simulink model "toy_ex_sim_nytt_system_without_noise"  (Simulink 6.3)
settings: Solver=ode4  StartTime=0.0  StopTime=simtid  FixedStep=.05  RelTol=1e-5
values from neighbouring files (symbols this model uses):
  alpha = -0.9    [bounds.m]    (also in real_ex_linkomb_W_and_DP.m = 1; real_ex_linkomb_W_and_RHOT.m = -0.2; real_ex_without_noise_z_30.m = -6:0.01:4; toy_ex_nytt_system.m)
  den_G1 = [-1 1]    [bounds.m]    (also in toy_ex_nytt_system.m; toy_ex_nytt_system_without_noise.m; toy_ex_nytt_system_with_disturbance.m; toy_ex_nytt_system_with_measure_noise.m)
  den_G2 = [-1 1]    [bounds.m]    (also in toy_ex_nytt_system.m; toy_ex_nytt_system_without_noise.m; toy_ex_nytt_system_with_disturbance.m; toy_ex_nytt_system_with_measure_noise.m)
  K_indre = 10    [real_ex_linkomb_W_and_DP.m]    (also in real_ex_linkomb_W_and_RHOT.m = 5; toy_ex_nytt_system.m = 50; toy_ex_nytt_system_without_noise.m = 20; toy_ex_nytt_system_with_disturbance.m = 50)
  K_ytre = 0.01    [real_ex_linkomb_W_and_DP.m]    (also in real_ex_linkomb_W_and_RHOT.m; toy_ex_nytt_system.m = 0.1; toy_ex_nytt_system_without_noise.m = 0.1; toy_ex_nytt_system_with_disturbance.m = 0.1)
  num_G1 = 5*[-1.5 1]    [bounds.m]    (also in toy_ex_nytt_system.m; toy_ex_nytt_system_without_noise.m; toy_ex_nytt_system_with_disturbance.m; toy_ex_nytt_system_with_measure_noise.m)
  num_G2 = 5*[-0.5 1]    [bounds.m]    (also in toy_ex_nytt_system.m; toy_ex_nytt_system_without_noise.m; toy_ex_nytt_system_with_disturbance.m; toy_ex_nytt_system_with_measure_noise.m)
  Ti = 100    [real_ex_linkomb_W_and_DP.m]    (also in real_ex_linkomb_W_and_RHOT.m = 100000; toy_ex_nytt_system.m = 10; toy_ex_nytt_system_without_noise.m = 10; toy_ex_nytt_system_with_disturbance.m = 10)

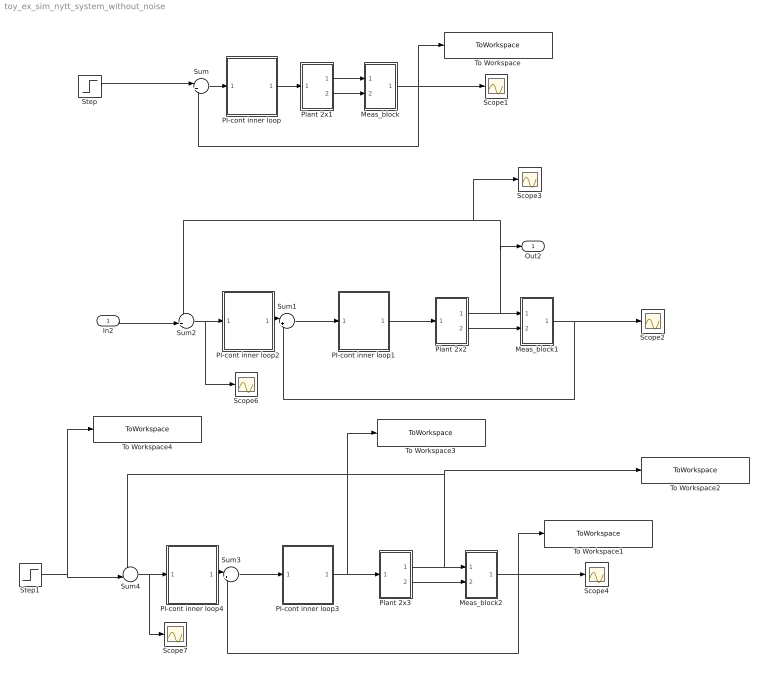
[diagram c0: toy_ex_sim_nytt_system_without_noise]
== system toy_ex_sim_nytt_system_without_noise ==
  In2 : Inport
  Meas_block : Subsystem
  Meas_block1 : Subsystem
  Meas_block2 : Subsystem
  PI-cont inner loop : Subsystem
  PI-cont inner loop1 : Subsystem
  PI-cont inner loop2 : Subsystem
  PI-cont inner loop3 : Subsystem
  PI-cont inner loop4 : Subsystem
  Plant 2x1 : Subsystem
  Plant 2x2 : Subsystem
  Plant 2x3 : Subsystem
  Scope{1..4,6..7} (6 alike) : Scope
  Step : Step  SampleTime=0
  Step1 : Step  Time=10  SampleTime=0
  Sum : Sum  Inputs=|+-
  Sum1 : Sum  Inputs=|+-
  Sum2 : Sum  Inputs=-+|
  Sum3 : Sum  Inputs=|+-
  Sum4 : Sum  Inputs=-+|
  To Workspace : ToWorkspace  VariableName=meas_linkomb  SampleTime=-1  SaveFormat=Structure With Time
  To Workspace1 : ToWorkspace  VariableName=meas_linkomb2  SampleTime=-1  SaveFormat=Structure With Time
  To Workspace2 : ToWorkspace  VariableName=meas_y1  SampleTime=-1  SaveFormat=Structure With Time
  To Workspace3 : ToWorkspace  VariableName=paadrag  SampleTime=-1  SaveFormat=Structure With Time
  To Workspace4 : ToWorkspace  VariableName=reference  SampleTime=-1  SaveFormat=Structure With Time
  Out2 : Outport
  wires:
  Plant 2x1/2(y2) -> Meas_block/2(In2)
  Plant 2x1/1("y1 ") -> Meas_block/1(In1)
  Meas_block/1(Out1) -> Scope1/1, To Workspace/1, Sum/2
  Sum/1 -> PI-cont inner loop/1(In1)
  PI-cont inner loop/1(Out1) -> Plant 2x1/1(In1)
  Plant 2x2/2(y2) -> Meas_block1/2(In2)
  Plant 2x2/1("y1 ") -> Meas_block1/1(In1), Out2/1, Sum2/1, Scope3/1
  Meas_block1/1(Out1) -> Scope2/1, Sum1/2
  Sum1/1 -> PI-cont inner loop1/1(In1)
  PI-cont inner loop1/1(Out1) -> Plant 2x2/1(In1)
  PI-cont inner loop2/1(Out1) -> Sum1/1
  Sum2/1 -> PI-cont inner loop2/1(In1), Scope6/1
  In2/1 -> Sum2/2
  Step/1 -> Sum/1
  Plant 2x3/2(y2) -> Meas_block2/2(In2)
  Plant 2x3/1("y1 ") -> Meas_block2/1(In1), To Workspace2/1, Sum4/1
  Meas_block2/1(Out1) -> Sum3/2, Scope4/1, To Workspace1/1
  Sum3/1 -> PI-cont inner loop3/1(In1)
  PI-cont inner loop3/1(Out1) -> Plant 2x3/1(In1), To Workspace3/1
  PI-cont inner loop4/1(Out1) -> Sum3/1
  Sum4/1 -> Scope7/1, PI-cont inner loop4/1(In1)
  Step1/1 -> Sum4/2, To Workspace4/1

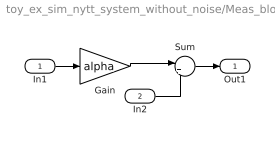
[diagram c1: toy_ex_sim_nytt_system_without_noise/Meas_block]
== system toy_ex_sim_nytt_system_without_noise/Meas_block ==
  In1 : Inport
  In2 : Inport  Port=2
  Gain : Gain  Gain=alpha
  Sum : Sum  Inputs=|++
  Out1 : Outport
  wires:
  Gain/1 -> Sum/1
  In1/1 -> Gain/1
  Sum/1 -> Out1/1
  In2/1 -> Sum/2

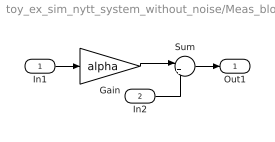
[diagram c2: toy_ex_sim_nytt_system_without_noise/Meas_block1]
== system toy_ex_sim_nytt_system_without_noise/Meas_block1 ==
  In1 : Inport
  In2 : Inport  Port=2
  Gain : Gain  Gain=alpha
  Sum : Sum  Inputs=|++
  Out1 : Outport
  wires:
  In2/1 -> Sum/2
  Sum/1 -> Out1/1
  In1/1 -> Gain/1
  Gain/1 -> Sum/1

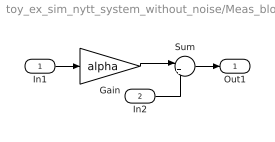
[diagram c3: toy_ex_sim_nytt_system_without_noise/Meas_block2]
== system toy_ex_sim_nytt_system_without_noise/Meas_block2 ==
  In1 : Inport
  In2 : Inport  Port=2
  Gain : Gain  Gain=alpha
  Sum : Sum  Inputs=|++
  Out1 : Outport
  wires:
  Gain/1 -> Sum/1
  In1/1 -> Gain/1
  Sum/1 -> Out1/1
  In2/1 -> Sum/2

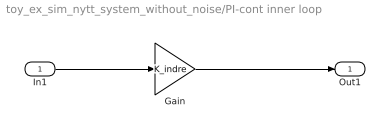
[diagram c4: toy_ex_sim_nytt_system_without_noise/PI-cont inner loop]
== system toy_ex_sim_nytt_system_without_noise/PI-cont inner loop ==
  In1 : Inport
  Gain : Gain  Gain=K_indre
  Out1 : Outport
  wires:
  Gain/1 -> Out1/1
  In1/1 -> Gain/1

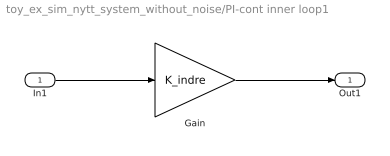
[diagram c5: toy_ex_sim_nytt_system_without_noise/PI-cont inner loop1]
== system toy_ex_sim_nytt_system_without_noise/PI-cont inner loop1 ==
  In1 : Inport
  Gain : Gain  Gain=K_indre
  Out1 : Outport
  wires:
  In1/1 -> Gain/1
  Gain/1 -> Out1/1

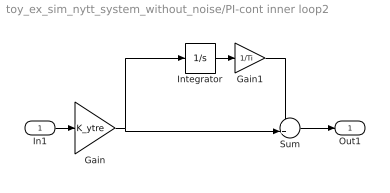
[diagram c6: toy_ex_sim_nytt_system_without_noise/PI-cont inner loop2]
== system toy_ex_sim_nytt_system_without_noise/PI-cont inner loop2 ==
  In1 : Inport
  Gain : Gain  Gain=K_ytre
  Gain1 : Gain  Gain=1/Ti
  Integrator : Integrator
  Sum : Sum  Inputs=++|
  Out1 : Outport
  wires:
  Gain/1 -> Integrator/1, Sum/2
  In1/1 -> Gain/1
  Integrator/1 -> Gain1/1
  Gain1/1 -> Sum/1
  Sum/1 -> Out1/1

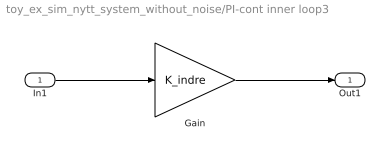
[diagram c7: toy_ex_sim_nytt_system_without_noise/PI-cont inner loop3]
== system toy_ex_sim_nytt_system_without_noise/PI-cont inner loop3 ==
  In1 : Inport
  Gain : Gain  Gain=K_indre
  Out1 : Outport
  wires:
  Gain/1 -> Out1/1
  In1/1 -> Gain/1

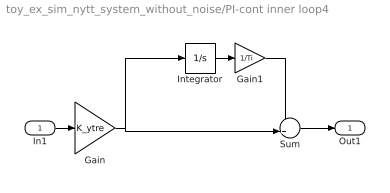
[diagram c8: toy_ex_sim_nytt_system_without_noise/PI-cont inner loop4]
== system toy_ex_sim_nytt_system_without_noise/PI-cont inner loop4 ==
  In1 : Inport
  Gain : Gain  Gain=K_ytre
  Gain1 : Gain  Gain=1/Ti
  Integrator : Integrator
  Sum : Sum  Inputs=++|
  Out1 : Outport
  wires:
  Sum/1 -> Out1/1
  Gain1/1 -> Sum/1
  Integrator/1 -> Gain1/1
  In1/1 -> Gain/1
  Gain/1 -> Sum/2, Integrator/1

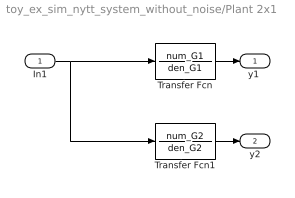
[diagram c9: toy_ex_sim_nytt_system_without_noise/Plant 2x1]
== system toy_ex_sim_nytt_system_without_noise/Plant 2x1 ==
  In1 : Inport
  Transfer Fcn : TransferFcn  Numerator=num_G1  Denominator=den_G1
  Transfer Fcn1 : TransferFcn  Numerator=num_G2  Denominator=den_G2
  "y1 " : Outport
  y2 : Outport  Port=2
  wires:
  In1/1 -> Transfer Fcn1/1, Transfer Fcn/1
  Transfer Fcn/1 -> "y1 "/1
  Transfer Fcn1/1 -> y2/1

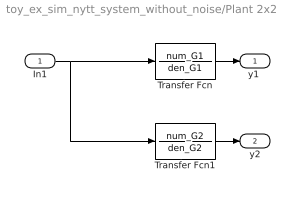
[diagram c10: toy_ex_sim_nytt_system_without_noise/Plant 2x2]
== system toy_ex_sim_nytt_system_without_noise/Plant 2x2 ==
  In1 : Inport
  Transfer Fcn : TransferFcn  Numerator=num_G1  Denominator=den_G1
  Transfer Fcn1 : TransferFcn  Numerator=num_G2  Denominator=den_G2
  "y1 " : Outport
  y2 : Outport  Port=2
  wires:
  Transfer Fcn1/1 -> y2/1
  Transfer Fcn/1 -> "y1 "/1
  In1/1 -> Transfer Fcn/1, Transfer Fcn1/1

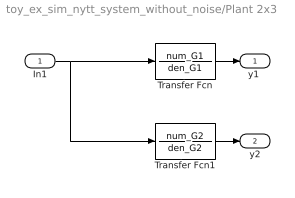
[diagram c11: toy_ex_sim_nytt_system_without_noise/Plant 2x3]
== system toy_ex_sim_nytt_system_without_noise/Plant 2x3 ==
  In1 : Inport
  Transfer Fcn : TransferFcn  Numerator=num_G1  Denominator=den_G1
  Transfer Fcn1 : TransferFcn  Numerator=num_G2  Denominator=den_G2
  "y1 " : Outport
  y2 : Outport  Port=2
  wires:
  In1/1 -> Transfer Fcn1/1, Transfer Fcn/1
  Transfer Fcn/1 -> "y1 "/1
  Transfer Fcn1/1 -> y2/1
